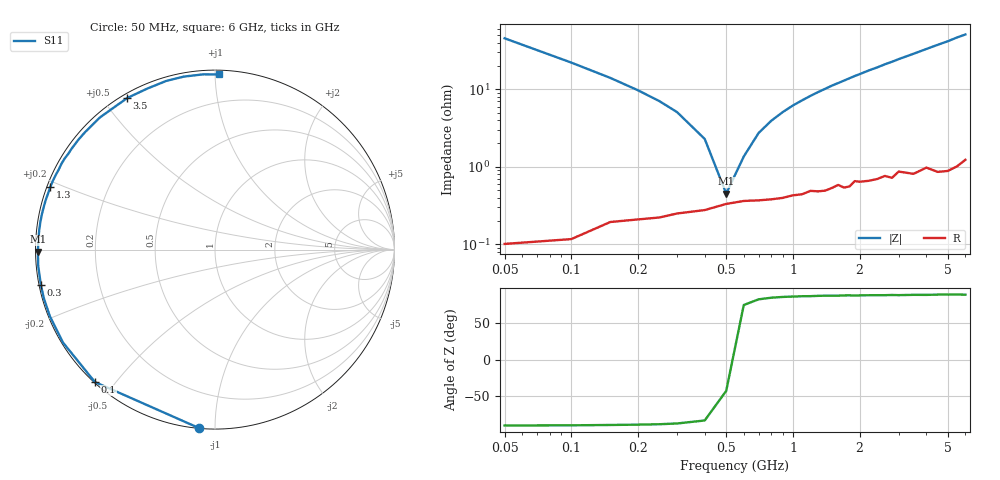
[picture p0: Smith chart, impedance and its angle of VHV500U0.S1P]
! Infineon Technologies  Discrete & RF Semiconductors
! BB 814
! Si Tuning Diode in SOT23
! VR = 0.5 V
! S-Parameters:  July  1999
# GHz  S  MA  R  50
!  f  S11
! GHz  MAG  ANG
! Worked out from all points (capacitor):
!   34 points, 50 MHz to 6 GHz, reference 50 ohm
!   read as one part to ground: C = 69.2 pF near 50 MHz
!   lowest |Z| = 451 mohm at 500 MHz (marker M1)
!   series resonance near 518.9 MHz, so ESL is about 1.4 nH
!   S11 on the Smith chart (normalised r, x): 50 MHz: 0.00, -0.91; 100 MHz: 0.00, -0.44; 300 MHz: 0.00, -0.10; 1.3 GHz: 0.01, +0.18; 3.5 GHz: 0.02, +0.58; 6 GHz: 0.02, +1.02
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0.05  0.9978 -95.2
0.1  0.9961 -132.2
0.15  0.9928 -148.6
0.2  0.992 -158.0
0.25  0.9913 -164.0
0.3  0.9902 -168.4
0.4  0.989 -174.8
0.5  0.9868 -179.3
0.6  0.9856 177.0
0.7  0.9854 173.8
0.8  0.985 171.0
1  0.9833 165.9
1.3  0.9815 159.1
1.5  0.9799 154.8
1.6  0.9782 152.9
1.8  0.9795 148.9
1.9  0.9763 146.9
2.2  0.9768 141.3
2.4  0.976 138.0
2.6  0.9744 134.3
2.8  0.9764 131.1
3  0.9724 127.7
3.5  0.9759 120.1
4  0.9733 112.8
4.5  0.9783 106.1
5  0.9794 100.2
5.5  0.9786 93.8
6  0.9762 88.7
